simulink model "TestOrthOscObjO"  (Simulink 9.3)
settings: Solver=FixedStepDiscrete  StartTime=0.0  StopTime=10000  FixedStep=Tstep  RelTol=1e-3  EnableMultiTasking=on
InitFcn:
  | TestOrthOscObjO.TestOrthOscObjO_init();
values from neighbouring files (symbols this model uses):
  Tfq = 0.020    (= 0.02)    [TestOrthOscObjO_init.m]    (also in TestOrthOsc_init.m)
  Tinit = 0.100    (= 0.1)    [TestOrthOscObjO_init.m]    (also in InspcCtrl_init.m = 0.001; TestOrthOsc_init.m = 0.001; Test_PIDctrl_init.m = 0.001; Test_LibVishia_Inspc_init.m = 0.002)
  Tstep = 0.0005    [TestOrthOscObjO_init.m]    (also in InspcCtrl_init.m = 0.0001; stimuli_Smlk.m = 0.001; TestOrthOsc_init.m = 5e-05; Test_PIDctrl_init.m = 0.0001)
undefined symbols (not defined in the file or in its folder): TestOrthi
libraries: libVishia_Conv x12, libVishia_CtrlSfn x12, libVishia_Inspc x7, libVishia_Ctrl x2, simulink x1

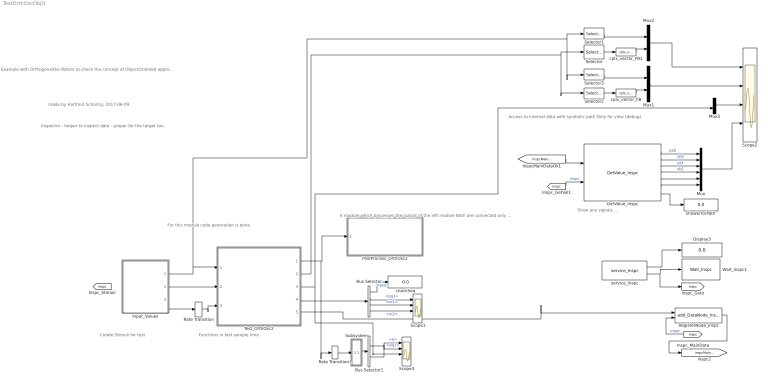
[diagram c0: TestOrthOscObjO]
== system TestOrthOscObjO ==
  note: ya0
  note: Inspector - helper to inspect data - proper for the target too.
  note: A module which processes the output of the left module Both are connected only via a handle in the Tinit time.
  note: Create Stimuli for test
  note: Show any signals ...
  note: made by Hartmut Schorrig, 2017-06-09
  note: Example with OrthogonalOscillators to check the concept of ObjectOriented approach in Simulink with handles to connect the Object-FB with the Operation-FB.
  note: Functions in fast sample time
  note: Access to internal data with symbolic path Only for view (debug)
  note: For this module code generation is done.
  Bus Selector : BusSelector  Commented=on  OutputSignals=seq,pq1,m1,m2
  Bus Selector1 : BusSelector  Commented=on  OutputSignals=e,pq1
  Display3 : Display
  GetValue_Inspc : libVishia_Inspc/GetValue_Inspc  Tstep=Tstep  path1='main_data.osc1[1].yab.re'  path2='main_data.osc1[1].yab.im'  path3='main_data.osc2[1].yab.re'  path4='main_data.osc2[1].yab.im'  path5='main_data.osc3[1].yab.re'  path6='main_data.osc3[1].yab.im'
  Input_Values : Subsystem
  Mux : Mux  Inputs=6
  Mux1 : Mux  Inputs=2
  Mux2 : Mux  Inputs=2
  Mux3 : Mux  Inputs=2
  PostProcess_OrthOsc2 : Subsystem  Commented=on  TreatAsAtomicUnit=on
  Rate Transition : RateTransition  Deterministic=off  OutPortSampleTime=Tfq
  Rate Transition1 : RateTransition  Deterministic=off  OutPortSampleTime=Tstep
  RegisterNode_Inspc : libVishia_Inspc/add_DataNode_Inspc  name1Refl='main'  name2Refl='_data'
  Scope1 : Scope  NumInputPorts=4
  Scope2 : Scope  NumInputPorts=4
  Scope3 : Scope  NumInputPorts=4
  Selector : Selector  IndexMode=Zero-based  InputPortWidth=2  IndexOptions=Index vector (dialog)  Indices=[0]  OutputSizes=1
  Selector1 : Selector  IndexMode=Zero-based  InputPortWidth=2  IndexOptions=Index vector (dialog)  Indices=[0]  OutputSizes=1
  Selector2 : Selector  IndexMode=Zero-based  InputPortWidth=2  IndexOptions=Index vector (dialog)  Indices=[1]  OutputSizes=1
  Selector3 : Selector  IndexMode=Zero-based  InputPortWidth=2  IndexOptions=Index vector (dialog)  Indices=[1]  OutputSizes=1
  Subsystem : Subsystem  Commented=on
  Test_OrthOsc2 : Subsystem  LoadFcn=TestOrthi.genBus();  TreatAsAtomicUnit=on
  Wait_Inspc1 : libVishia_Inspc/Wait_Inspc  Commented=on  Tstep=Tstep  cyclesStart=9999999  delay_ms=0
  checkSeq : Display
  cplx_vector_FB : libVishia_Conv/cplx_vector_FB  SystemSampleTime=-1
  cplx_vector_FB1 : libVishia_Conv/cplx_vector_FB  SystemSampleTime=-1
  service_Inspc : libVishia_Inspc/service_Inspc  Tstep=Tstep  IpPort='UDP:0.0.0.0:60094'
  showErrorPath : Display
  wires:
  Mux2/1 -> Scope2/1
  Test_OrthOsc2/3(ypq) -> Mux3/2, Scope3/3
  Input_Values/3(Out3) -> Rate Transition/1
  Input_Values/1(Out1) -> Selector3/1, Selector1/1, Test_OrthOsc2/1(x)
  Input_Values/2(Out2) -> Test_OrthOsc2/2(wi)
  Test_OrthOsc2/2(ypq2) -> Selector2/1, Selector/1
  cplx_vector_FB1/1 -> Mux2/2
  Selector/1 -> cplx_vector_FB1/1
  Test_OrthOsc2/1(ya3) -> Rate Transition1/1, PostProcess_OrthOsc2/1(In1)
  Selector1/1 -> Mux2/1
  cplx_vector_FB/1 -> Mux1/2
  Selector2/1 -> cplx_vector_FB/1
  Selector3/1 -> Mux1/1
  Mux1/1 -> Scope2/2
  [inspc] -> RegisterNode_Inspc/2  "inspc"
  Test_OrthOsc2/5(data_inspc) -> RegisterNode_Inspc/1
  [inspc] -> GetValue_Inspc/2  "inspc"
  Mux/1 -> Scope2/4
  GetValue_Inspc/7 -> showErrorPath/1
  GetValue_Inspc/1 -> Mux/1
  GetValue_Inspc/2 -> Mux/2  "yb0"
  GetValue_Inspc/3 -> Mux/3  "ya1"
  GetValue_Inspc/4 -> Mux/4  "yb1"
  GetValue_Inspc/6 -> Mux/6
  GetValue_Inspc/5 -> Mux/5
  Mux3/1 -> Scope2/3
  RegisterNode_Inspc/1 -> [inspcMainDataOk]
  [inspc] -> ?  "inspc"
  [inspcMainDataOk] -> GetValue_Inspc/1
  service_Inspc/2 -> Wait_Inspc1/1, [inspc]
  Rate Transition/1 -> Test_OrthOsc2/3(fq)
  Bus Selector/2 -> Scope1/1  "<pq1>"
  Bus Selector/3 -> Scope1/2  "<m1>"
  Bus Selector/4 -> Scope1/3  "<m2>"
  Bus Selector/1 -> checkSeq/1  "<seq>"
  Test_OrthOsc2/4(ya1) -> Bus Selector/1
  Rate Transition1/1 -> Subsystem/1(In1)
  Subsystem/1(Out1) -> Bus Selector1/1
  Bus Selector1/1 -> Scope3/1  "<e>"
  Bus Selector1/2 -> Scope3/2  "<pq1>"
  service_Inspc/1 -> Display3/1

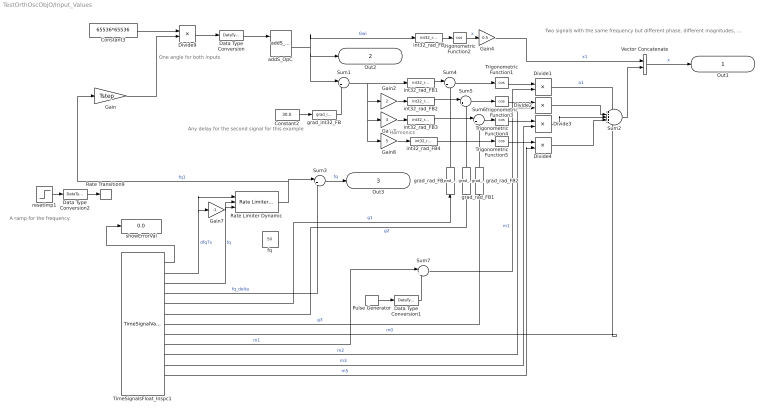
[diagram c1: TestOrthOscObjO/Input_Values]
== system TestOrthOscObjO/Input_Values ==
  note: A ramp for the frequency
  note: Two signals with the same frequency but different phase, different magnitudes, one signal has harmonics.
  note: Harmonics
  note: Any delay for the second signal for this example
  note: One angle for both inputs
  Constant2 : Constant  Value=30.0  OutDataTypeStr=single
  Constant3 : Constant  Value=65536*65536  OutDataTypeStr=single
  Data Type Conversion : DataTypeConversion  OutDataTypeStr=int32
  Data Type Conversion1 : DataTypeConversion  OutDataTypeStr=single
  Data Type Conversion2 : DataTypeConversion  OutDataTypeStr=single
  Divide{1..4,9} (5 alike) : Product  Inputs=**
  Gain : Gain  Gain=Tstep
  Gain2 : Gain  Gain=2
  Gain3 : Gain  Gain=3
  Gain4 : Gain  Gain=0.5
  Gain7 : Gain  Gain=-1
  Gain8 : Gain  Gain=5
  Pulse Generator : DiscretePulseGenerator  PulseType=Time based  Amplitude=0.2  Period=1  PulseWidth=40
  Rate Limiter Dynamic : simulink/Discontinuities/Rate Limiter Dynamic
  Rate Transition9 : RateTransition  Integrity=off  Deterministic=off  OutPortSampleTime=Tfq
  Sum{1,3..7} (6 alike) : Sum  Inputs=|++
  Sum2 : Sum  Inputs=+++++
  TimeSignalsFloat_Inspc1 : libVishia_Inspc/TimeSignalValue_Inspc  Description=|  Tstep=Tstep  filepath=timeSignalFilepath  nameRefl='stimuli'  nrofStimuli=25  varDef=|
      | A combined stimuli and inspector function block.
      | Stimuli file path: file contains stimuli in form:
      |   %time:0: stimuli.namex = 5000.0, stimuli.namey = 50.0 -10; 
      | Name in reflection-tree: Name of this function block for stimuli and inspector access
      | name1..12: output type and name, base type is single always.
      | C2:namexy  A complex array of 2 elements
      | 6:namexy An array of 6 elements (max).
      | C:namexy  A 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
      | dfq7s:F;
      | fq:F;
      | fq_delta:F;
      | g1:F;
      | g2:F;
      | g3:F;
      | m0:F;
      | m1:F;
      | m2:F;
      | m3:F;
      | m5:F;
  Trigonometric Function{1..5} (5 alike) : Trigonometry  Operator=cos
  Vector Concatenate : Concatenate
  addS_OpC : libVishia_Ctrl/addS_OpC  init=0  Tstep=-1
  fq : Constant  Value=50  OutDataTypeStr=single
  grad_int32_FB : libVishia_Conv/grad_int32_FB  SystemSampleTime=-1
  grad_rad_FB : libVishia_Conv/grad_rad_FB  SystemSampleTime=-1
  grad_rad_FB1 : libVishia_Conv/grad_rad_FB  SystemSampleTime=-1
  grad_rad_FB2 : libVishia_Conv/grad_rad_FB  SystemSampleTime=-1
  int32_rad_FB{,1..4} (5 alike) : libVishia_Conv/int32_rad_FB  SystemSampleTime=-1
  resetImp1 : Step  Time=0.1  Before=0.995  After=1.2  SampleTime=Tfq
  showErrorVal : Display
  Out1 : Outport  OutDataTypeStr=single  PortDimensions=2
  Out2 : Outport  Port=2  OutDataTypeStr=int32  PortDimensions=1
  Out3 : Outport  Port=3  OutDataTypeStr=single  PortDimensions=1
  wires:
  TimeSignalsFloat_Inspc1/4 -> Sum3/2  "fq_delta"
  Constant3/1 -> Divide9/1
  int32_rad_FB/1 -> Trigonometric Function2/1
  Trigonometric Function2/1 -> Gain4/1  "x"
  Divide9/1 -> Data Type Conversion/1
  int32_rad_FB1/1 -> Sum4/1
  Trigonometric Function1/1 -> Divide1/1
  Constant2/1 -> grad_int32_FB/1
  Gain4/1 -> Vector Concatenate/1  "x1"
  Divide1/1 -> Sum2/1  "a1"
  Gain/1 -> Divide9/2
  Data Type Conversion/1 -> addS_OpC/1
  Data Type Conversion2/1 -> Rate Transition9/1
  Gain3/1 -> int32_rad_FB3/1
  Gain2/1 -> int32_rad_FB2/1
  int32_rad_FB2/1 -> Sum5/1
  int32_rad_FB3/1 -> Sum6/1
  Trigonometric Function3/1 -> Divide2/1
  Divide2/1 -> Sum2/2
  Trigonometric Function4/1 -> Divide3/1
  Divide3/1 -> Sum2/3
  Sum2/1 -> Vector Concatenate/2
  Rate Transition9/1 -> ?
  resetImp1/1 -> Data Type Conversion2/1
  grad_int32_FB/1 -> Sum1/2
  Vector Concatenate/1 -> Out1/1  "x"
  addS_OpC/2 -> int32_rad_FB/1, Sum1/1, Out2/1  "Gwi"
  Sum7/1 -> Divide1/2  "m1"
  TimeSignalsFloat_Inspc1/10 -> Divide2/2  "m2"
  TimeSignalsFloat_Inspc1/11 -> Divide3/2  "m3"
  Sum6/1 -> Trigonometric Function4/1
  TimeSignalsFloat_Inspc1/5 -> grad_rad_FB/1  "g1"
  TimeSignalsFloat_Inspc1/6 -> grad_rad_FB1/1  "g2"
  TimeSignalsFloat_Inspc1/7 -> grad_rad_FB2/1  "g3"
  Sum5/1 -> Trigonometric Function3/1
  Sum4/1 -> Trigonometric Function1/1
  grad_rad_FB/1 -> Sum4/2
  grad_rad_FB1/1 -> Sum5/2
  grad_rad_FB2/1 -> Sum6/2
  Rate Limiter Dynamic/1 -> Sum3/1, Gain/1  "fq1"
  TimeSignalsFloat_Inspc1/3 -> Rate Limiter Dynamic/2  "fq"
  Sum3/1 -> Out3/1  "fq"
  TimeSignalsFloat_Inspc1/2 -> Gain7/1, Rate Limiter Dynamic/1  "dfq7s"
  Gain7/1 -> Rate Limiter Dynamic/3
  Sum1/1 -> int32_rad_FB1/1, Gain8/1, Gain3/1, Gain2/1
  Gain8/1 -> int32_rad_FB4/1
  Trigonometric Function5/1 -> Divide4/1
  Divide4/1 -> Sum2/4
  int32_rad_FB4/1 -> Trigonometric Function5/1
  TimeSignalsFloat_Inspc1/12 -> Divide4/2  "m5"
  TimeSignalsFloat_Inspc1/8 -> Sum2/5  "m0"
  TimeSignalsFloat_Inspc1/1 -> showErrorVal/1
  Data Type Conversion1/1 -> Sum7/2
  TimeSignalsFloat_Inspc1/9 -> Sum7/1  "m1"
  Pulse Generator/1 -> Data Type Conversion1/1

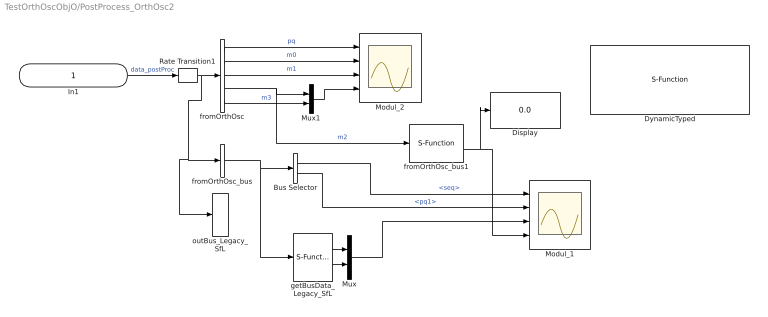
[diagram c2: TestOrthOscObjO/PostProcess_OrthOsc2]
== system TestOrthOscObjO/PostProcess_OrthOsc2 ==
  In1 : Inport  OutDataTypeStr=uint32
  Bus Selector : BusSelector  OutputSignals=seq,pq1
  Display : Display
  DynamicTyped : S-Function  Commented=on  FunctionName=getLocked_Output_Test_OrthOsc2_SfH  SFunctionDeploymentMode=off  EnableBusSupport=off
  Modul_1 : Scope  NumInputPorts=4
  Modul_2 : Scope  NumInputPorts=4
  Mux : Mux  Inputs=2
  Mux1 : Mux  Inputs=2
  Rate Transition1 : RateTransition  Integrity=off  OutPortSampleTime=Tfq
  fromOrthOsc : S-Function  FunctionName=getLocked_Output_Test_OrthOsc2_SfH  SFunctionDeploymentMode=off  EnableBusSupport=off
  fromOrthOsc_bus : S-Function  FunctionName=getSyncBus_Output_Test_OrthOsc2_SfH  SFunctionDeploymentMode=off  EnableBusSupport=off
  fromOrthOsc_bus1 : S-Function  FunctionName=step_Test_ArrayVoid_SmlkObjO_SfH  SFunctionDeploymentMode=off  EnableBusSupport=off
  getBusData_Legacy_SfL : S-Function  FunctionName=getBusData_Legacy_SfL  SFunctionDeploymentMode=off  EnableBusSupport=off
  outBus_Legacy_SfL : S-Function  FunctionName=outBus_Legacy_SfL  SFunctionDeploymentMode=off  EnableBusSupport=off
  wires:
  In1/1 -> Rate Transition1/1  "data_postProc"
  fromOrthOsc/2 -> Modul_2/2  "m0"
  fromOrthOsc/4 -> fromOrthOsc_bus1/1, Mux1/1  "m2"
  fromOrthOsc/5 -> Mux1/2  "m3"
  fromOrthOsc/1 -> Modul_2/1  "pq"
  Rate Transition1/1 -> outBus_Legacy_SfL/1, fromOrthOsc_bus/1, fromOrthOsc/1
  Mux1/1 -> Modul_2/4
  fromOrthOsc/3 -> Modul_2/3  "m1"
  fromOrthOsc_bus/1 -> getBusData_Legacy_SfL/1, Bus Selector/1
  Bus Selector/1 -> Modul_1/1  "<seq>"
  Bus Selector/2 -> Modul_1/2  "<pq1>"
  getBusData_Legacy_SfL/1 -> Mux/1
  getBusData_Legacy_SfL/2 -> Mux/2
  Mux/1 -> Modul_1/3
  fromOrthOsc_bus1/2 -> Display/1, Modul_1/4

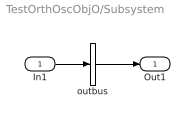
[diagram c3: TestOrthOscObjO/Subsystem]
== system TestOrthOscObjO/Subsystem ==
  In1 : Inport
  outbus : S-Function  FunctionName=getBus_Output_Test_OrthOsc2_SfH  SFunctionDeploymentMode=off  EnableBusSupport=off
  Out1 : Outport  OutDataTypeStr=Bus: Data_Output_Test_OrthOsc2
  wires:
  In1/1 -> outbus/1
  outbus/1 -> Out1/1

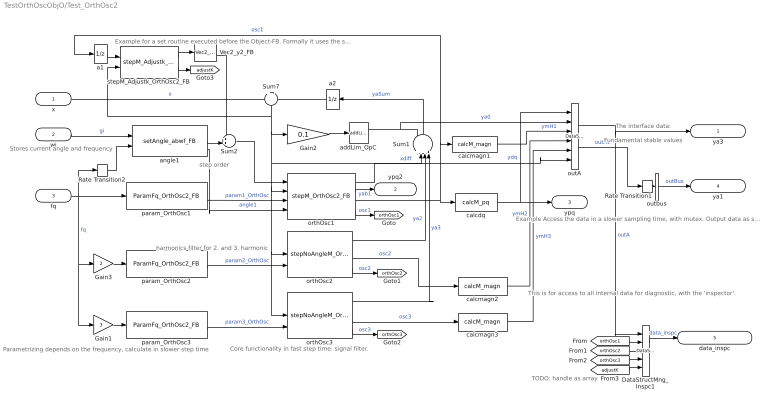
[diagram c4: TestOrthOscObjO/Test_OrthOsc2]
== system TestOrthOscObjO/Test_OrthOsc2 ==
  note: TODO: handle as array
  note: Example Access the data in a slower sampling time, with mutex. Output data as simulink bus
  note: The interface data:
  note: This is for access to all internal data for diagnostic, with the 'inspector'.
  note: Fundamental stable values
  note: harmonics filter for 2. and 3, harmonic
  note: Core functionality in fast step time: signal filter.
  note: Parametrizing depends on the frequency, calculate in slower step time
  note: Stores current angle and frequency
  note: Example for a set routine executed before the Object-FB. Formally it uses the stored thiz-reference from the last step time.
  note: step order
  x : Inport  OutDataTypeStr=single  PortDimensions=2  SampleTime=Tstep
  wi : Inport  Port=2  OutDataTypeStr=int32  SampleTime=Tstep
  fq : Inport  Port=3  OutDataTypeStr=single  SampleTime=Tfq
  DataStructMng_Inspc1 : libVishia_Inspc/DataStructMng_Inspc  Commented=on  dirGenSource=''  typeData='OrthOsc_Module'  inherit=off  chain=off  inputs=|
      | d: OrthOsc_Data;
      | =orthH1: OrthOsc2_FB_CtrlemC;
      | =orthH2: OrthOsc2_FB_CtrlemC;
      | =orthH3: OrthOsc2_FB_CtrlemC;
      | =adj: Adjustk_OrthOsc2_FB;
  Gain1 : Gain  Gain=3
  Gain2 : Gain  Gain=0.1
  Gain3 : Gain  Gain=2
  Rate Transition1 : RateTransition  Integrity=off  Deterministic=off  OutPortSampleTime=Tfq
  Rate Transition2 : RateTransition  Integrity=off  Deterministic=off  OutPortSampleTime=Tstep
  Sum1 : Sum  Inputs=++++|
  Sum2 : Sum  Inputs=++|
  Sum7 : Sum  Inputs=+|-
  Vec2_y2_FB : libVishia_Conv/Vec2_y2_FB  SystemSampleTime=-1
  a1 : UnitDelay  SampleTime=Tstep  HasFrameUpgradeWarning=on
  a2 : UnitDelay  SampleTime=Tstep  HasFrameUpgradeWarning=on
  addLim_OpC : libVishia_Ctrl/addLim_OpC  y0=0  lim=0.4
  angle1 : libVishia_CtrlSfn/setAngle_abwf_FB  identObj=16  Tstep=Tstep
  calcdq : libVishia_CtrlSfn/calcM_pq  SystemSampleTime=-1
  calcmagn1 : libVishia_CtrlSfn/calcM_magn  SystemSampleTime=-1
  calcmagn2 : libVishia_CtrlSfn/calcM_magn  SystemSampleTime=-1
  calcmagn3 : libVishia_CtrlSfn/calcM_magn  SystemSampleTime=-1
  orthOsc1 : libVishia_CtrlSfn/stepM_OrthOsc2_FB  ident=[21 22]  kA=2.0  kB=-2.0
  orthOsc2 : libVishia_CtrlSfn/stepNoAngleM_OrthOsc2_FB  ident=[31 32]  kA=0.3  kB=-0.3
  orthOsc3 : libVishia_CtrlSfn/stepNoAngleM_OrthOsc2_FB  ident=[41 42]  kA=0.3  kB=-0.3
  outA : libVishia_Inspc/DataStructMng_Inspc  dirGenSource=''  typeData='OrthOsc_Data'  inherit=off  chain=off  inputs=|
      | ypq: f*2;
      | ya0: F*2;
      | ymH1: F*2;
      | ymH2: F*2;
      | ymH3: F*2;
      | error: F*2;
  outbus : S-Function  Commented=on  FunctionName=getSyncBus_Output_Test_OrthOsc2_SfH  SFunctionDeploymentMode=off  EnableBusSupport=off
  param_OrthOsc1 : libVishia_CtrlSfn/ParamFq_OrthOsc2_FB  identObj=17  Tstep=Tfq  TstepOrth=Tstep  m_nom=1
  param_OrthOsc2 : libVishia_CtrlSfn/ParamFq_OrthOsc2_FB  identObj=18  Tstep=Tfq  TstepOrth=Tstep  m_nom=1
  param_OrthOsc3 : libVishia_CtrlSfn/ParamFq_OrthOsc2_FB  identObj=19  Tstep=Tfq  TstepOrth=Tstep  m_nom=1
  stepM_Adjustk_OrthOsc2_FB : libVishia_CtrlSfn/stepM_Adjustk_OrthOsc2_FB  ident=[21 22]  max_e=0.05  kHi=5  kNormal=2  Tdecay=0.1  Tstep=Tstep
  ya3 : Outport  OutDataTypeStr=uint32  SampleTime=Tinit
  ypq2 : Outport  Port=2  OutDataTypeStr=single  PortDimensions=2  SampleTime=Tstep
  ypq : Outport  Port=3  OutDataTypeStr=single  PortDimensions=2  SampleTime=Tstep
  ya1 : Outport  Port=4  OutDataTypeStr=Bus: Data_Output_Test_OrthOsc2
  data_inspc : Outport  Port=5  OutDataTypeStr=uint32  SampleTime=Tinit
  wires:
  fq/1 -> Rate Transition2/1, Gain1/1, Gain3/1, param_OrthOsc1/1  "fq"
  param_OrthOsc1/2 -> orthOsc1/3  "param1_OrthOsc"
  x/1 -> Sum7/1  "x"
  a2/1 -> Sum7/2
  wi/1 -> angle1/1  "gi"
  Sum1/1 -> a2/1  "yaSum"
  angle1/3 -> orthOsc1/4  "angle1"
  Gain3/1 -> param_OrthOsc2/1
  Gain1/1 -> param_OrthOsc3/1
  param_OrthOsc2/2 -> orthOsc2/3  "param2_OrthOsc"
  param_OrthOsc3/2 -> orthOsc3/3  "param3_OrthOsc"
  orthOsc2/1 -> Sum1/3  "ya2"
  orthOsc3/1 -> Sum1/4  "ya3"
  calcdq/1 -> ypq/1, outA/1  "ydq"
  Sum7/1 -> orthOsc3/2, orthOsc2/2, orthOsc1/2, outA/6, Gain2/1, stepM_Adjustk_OrthOsc2_FB/2  "xdiff"
  Rate Transition2/1 -> angle1/2
  orthOsc1/2 -> ypq2/1  "yab1"
  calcmagn2/1 -> outA/4  "ymH2"
  calcmagn3/1 -> outA/5  "ymH3"
  outA/1 -> DataStructMng_Inspc1/1, ya3/1  "outA"
  DataStructMng_Inspc1/1 -> data_inspc/1  "data_inspc"
  calcmagn1/1 -> outA/3  "ymH1"
  orthOsc1/3 -> a1/1, calcmagn1/1, calcdq/1  "osc1"
  orthOsc2/3 -> calcmagn2/1  "osc2"
  orthOsc3/3 -> calcmagn3/1  "osc3"
  orthOsc1/1 -> Sum1/2
  addLim_OpC/1 -> Sum1/1, outA/2  "ya0"
  Gain2/1 -> addLim_OpC/1
  angle1/2 -> Sum2/2
  outbus/1 -> ya1/1  "outBus"
  outA/2 -> Rate Transition1/1  "outA1"
  Rate Transition1/1 -> outbus/1
  a1/1 -> stepM_Adjustk_OrthOsc2_FB/1
  Sum2/1 -> orthOsc1/1
  stepM_Adjustk_OrthOsc2_FB/1 -> Vec2_y2_FB/1
  Vec2_y2_FB/2 -> Sum2/1
  orthOsc1/4 -> [orthOsc1]  "osc1"
  orthOsc2/4 -> [orthOsc2]  "osc2"
  orthOsc3/4 -> [orthOsc3]  "osc3"
  stepM_Adjustk_OrthOsc2_FB/2 -> [adjustK]
  [orthOsc1] -> DataStructMng_Inspc1/2
  [orthOsc2] -> DataStructMng_Inspc1/3
  [orthOsc3] -> DataStructMng_Inspc1/4
  [adjustK] -> DataStructMng_Inspc1/5
